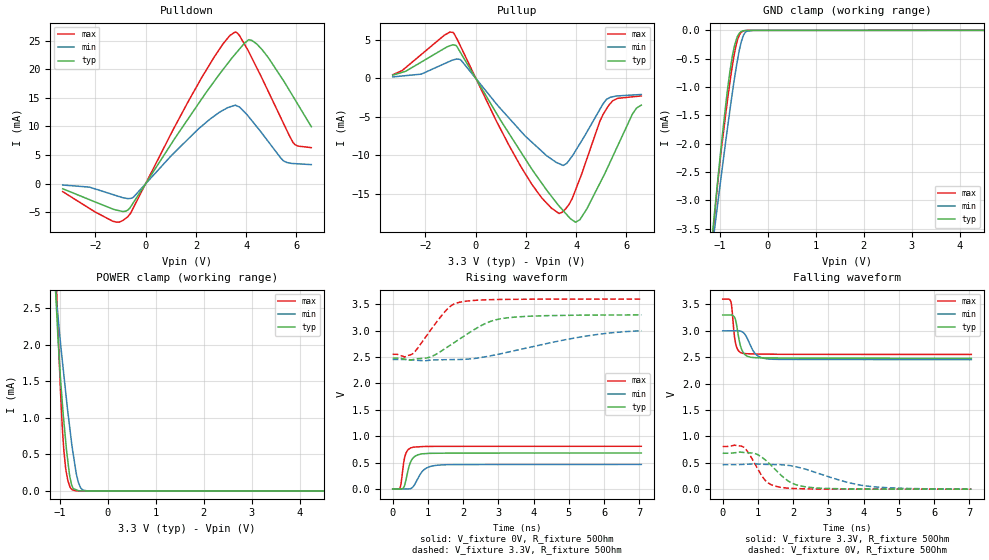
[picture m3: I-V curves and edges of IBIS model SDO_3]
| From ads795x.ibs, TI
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|   3-state SDO model 3V
[Model]   SDO_3
Model_type   3-state
|Signals   SDO
Vmeas = 1.65
Vref = 1.65
Cref = 15pF
Rref = 50
| variable   typ   min   max
|C_comp Output in tri-state
C_comp   8.5896378e-13   1.0282738e-12   6.9643676e-13
|C_comp Output High
|C_comp   8.0761158e-11   2.9350463e-11   1.7361130e-10
|C_comp Output Low
|C_comp   3.4327542e-11   1.3562603e-11   8.1374077e-11
[Voltage Range]   3.3   3   3.6
[Temperature Range]   27   125   -40
[Pullup Reference]   3.3   3   3.6
[Pulldown Reference]   0   0   0
[Power Clamp Reference]   3.3   3   3.6
[GND Clamp Reference]   0   0   0
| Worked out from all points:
|   slope of the pulldown table from 0 to 0.495 V, typ, clamps not added: 147 ohm
|   slope of the pullup table from 0 to 0.495 V, typ, clamps not added: 181 ohm
|   GND clamp passes 1 mA (typ) near -0.83 V on its own axis
|   POWER clamp passes 1 mA (typ) near -0.92 V on its own axis
|   falling waveform, V_fixture 3.3V, R_fixture 50Ohm: 20-80 % time 153ps typ, 258ps min, 101ps max; typ from 3.3 V to 2.48 V
|   rising waveform, V_fixture 0V, R_fixture 50Ohm: 20-80 % time 169ps typ, 274ps min, 111ps max; typ from 0 V to 0.681 V
|   rising waveform, V_fixture 3.3V, R_fixture 50Ohm: 20-80 % time 1.18ns typ, 2.35ns min, 712ps max; typ from 2.48 V to 3.3 V
|   falling waveform, V_fixture 0V, R_fixture 50Ohm: 20-80 % time 679ps typ, 1.4ns min, 444ps max; typ from 0.681 V to 0 V
[Pulldown]
|   Voltage   I(typ)   I(min)   I(max)
-3.3V     -901.2uA   -242.5uA   -1.4mA
-1.328V   -4.42mA    -1.879mA   -6.536mA
-730mV    -4.667mA   -2.602mA   -5.877mA
-483.5mV  -3.291mA   -2.355mA   -4.179mA
2.209V    14.69mA    9.99mA     18.4mA
3.087V    20.02mA    12.87mA    24.52mA
3.549V    22.6mA     13.71mA    26.52mA
4.092V    25.18mA    11.75mA    23.17mA
4.428V    24.41mA    9.923mA    20.22mA
5.477V    18.05mA    4.007mA    10.6mA
5.864V    15.26mA    3.521mA    7.19mA
6.59V     9.958mA    3.325mA    6.296mA
[GND Clamp]
|   Voltage   I(typ)   I(min)   I(max)
-3.3V     -23.43mA   -19.05mA   -29.08mA
-1.158V   -3.628mA   -3.832mA   -3.747mA
-1.11V    -3.214mA   -3.504mA   -3.279mA
-1.098V   -3.106mA   -3.418mA   -3.158mA
-971.9mV  -2.045mA   -2.574mA   -2.124mA
-789.1mV  -716.8uA   -1.398mA   -908.5uA
-736.3mV  -439.2uA   -1.084mA   -605.9uA
-669.1mV  -197.8uA   -707.1uA   -290.5uA
-558.3mV  -22.99uA   -218.5uA   -36.17uA
-473.3mV  -4.293uA   -39.69uA   -5.016uA
-312.7mV  -655.1nA   -464.5nA   -780.9nA
6.59V     0A         0A         0A
[Pullup]
|   Voltage   I(typ)   I(min)   I(max)
-3.3V     432.2uA    202.9uA    487.2uA
-1.246V   3.912mA    1.921mA    5.632mA
-789.1mV  4.304mA    2.506mA    5.42mA
1.323V    -7.139mA   -5.143mA   -8.687mA
2.621V    -13.6mA    -9.447mA   -15.52mA
3.322V    -16.62mA   -11.09mA   -17.57mA
3.627V    -17.74mA   -11.05mA   -16.77mA
3.969V    -18.71mA   -9.443mA   -14.55mA
4.931V    -13.71mA   -4.084mA   -5.654mA
5.281V    -11.37mA   -2.583mA   -3.562mA
6.234V    -4.651mA   -2.157mA   -2.391mA
6.59V     -3.471mA   -2.087mA   -2.272mA
[POWER Clamp]
|   Voltage   I(typ)   I(min)   I(max)
-3.3V     43.35mA    34.07mA    53.59mA
-1.085V   2.678mA    2.71mA     3.07mA
-1.07V    2.497mA    2.604mA    2.805mA
-988.9mV  1.559mA    2.041mA    1.393mA
-954.5mV  1.255mA    1.82mA     931.7uA
-917.8mV  957.3uA    1.593mA    562uA
-878.9mV  682.6uA    1.353mA    309.5uA
-833.1mV  403.4uA    1.077mA    140.9uA
-744mV    66.14uA    598.2uA    15.4uA
-613.9mV  2.958uA    116.7uA    1.254uA
-434.8mV  1.003uA    1.172uA    1.223uA
6.59V     0A         0A         0A
[Ramp]
R_load = 50
|   typ   min   max
dV/dt_r   0.408362/1.69045e-010  0.278215/2.69574e-010  0.484871/1.1023e-010
dV/dt_f   0.49235/1.52668e-010  0.327672/2.57441e-010  0.628238/1.00738e-010
[Falling Waveform]
V_fixture = 3.3V
V_fixture_min = 3V
V_fixture_max = 3.6V
R_fixture = 50Ohm
C_fixture = 0F
|   Time   V(typ)   V(min)   V(max)
0s        3.3V       3V         3.6V
226.8ps   3.3V       3V         3.561V
263.9ps   3.297V     3V         3.403V
327.8ps   3.266V     3V         2.927V
368.7ps   3.194V     3V         2.756V
478.9ps   2.781V     2.998V     2.602V
564.6ps   2.612V     2.978V     2.574V
922.4ps   2.492V     2.567V     2.561V
1.263ns   2.487V     2.469V     2.558V
7.054ns   2.479V     2.454V     2.553V
[Rising Waveform]
V_fixture = 0V
V_fixture_min = 0V
V_fixture_max = 0V
R_fixture = 50Ohm
C_fixture = 0F
|   Time   V(typ)   V(min)   V(max)
0s        -121.8nV   -126.6nV   -107.8nV
208.5ps   -2.699mV   -910.3uV   21.61mV
241.6ps   -3.128mV   -1.055mV   121.8mV
304.5ps   18.49mV    -1.329mV   461.3mV
398.8ps   240mV      -1.741mV   708mV
492.3ps   485.9mV    2.574mV    770.2mV
584.1ps   590.1mV    44.92mV    790.9mV
881.9ps   666.7mV    360.2mV    803.7mV
1.272ns   675.6mV    449.3mV    806.4mV
7.054ns   680.6mV    463.7mV    808.1mV
[Rising Waveform]
V_fixture = 3.3V
V_fixture_min = 3V
V_fixture_max = 3.6V
R_fixture = 50Ohm
C_fixture = 0F
|   Time   V(typ)   V(min)   V(max)
0s        2.479V     2.454V     2.553V
332.1ps   2.461V     2.454V     2.5V
574.5ps   2.452V     2.445V     2.567V
1.069ns   2.501V     2.441V     3.005V
1.512ns   2.672V     2.45V      3.384V
1.894ns   2.841V     2.454V     3.54V
2.669ns   3.149V     2.51V      3.586V
3.14ns    3.235V     2.574V     3.594V
5.422ns   3.295V     2.891V     3.599V
7.054ns   3.3V       3V         3.6V
[Falling Waveform]
|Gnd
V_fixture = 0V
V_fixture_min = 0V
V_fixture_max = 0V
R_fixture = 50Ohm
C_fixture = 0F
|   Time   V(typ)   V(min)   V(max)
0s        680.6mV    463.7mV    808.1mV
593.3ps   695.2mV    469.6mV    795.3mV
963.3ps   664mV      477.1mV    419.9mV
1.202ns   557.8mV    470.1mV    170.1mV
1.617ns   288.3mV    464.6mV    37.88mV
1.968ns   113mV      439.5mV    14mV
2.595ns   26.36mV    325.5mV    2.504mV
3.531ns   4.19mV     130.2mV    1.979mV
4.23ns    1.554mV    48.29mV    1.586mV
7.054ns   -121.8nV   -126.6nV   -107.8nV
